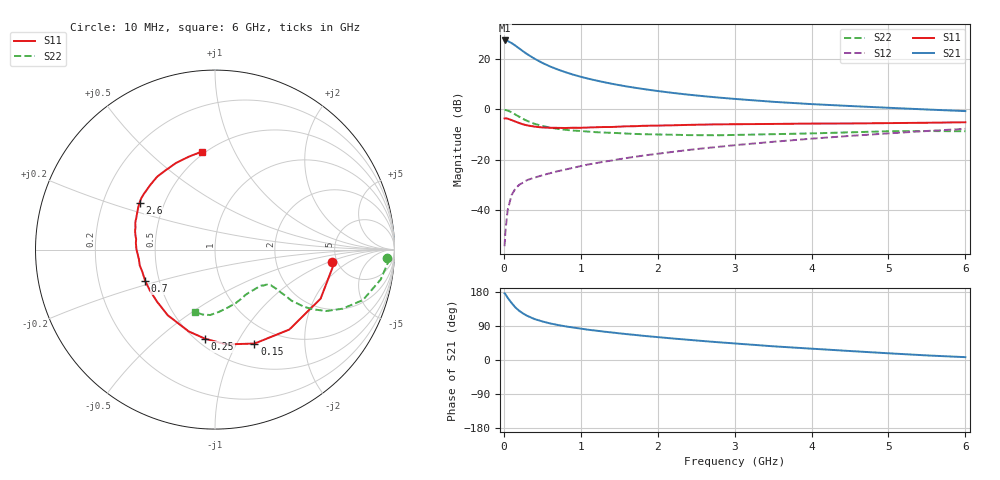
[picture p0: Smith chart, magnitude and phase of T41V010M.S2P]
! Infineon Technologies  Discrete & RF Semiconductors
! BFR182T
! Si NPN RF Bipolar Junction Transistor in SC75
! VCE = 1 V  IC = 10 mA
! Common Emitter S-Parameters:  October  1999
# GHz  S  MA  R  50
!  f  S11  S21  S12  S22
! GHz  MAG  ANG  MAG  ANG  MAG  ANG  MAG  ANG
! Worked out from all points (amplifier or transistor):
!   36 points, 10 MHz to 6 GHz, reference 50 ohm
!   highest |S21| = 27.3 dB at 10 MHz (marker M1)
!   |S21| within 3 dB of that: start of sweep to 192.3 MHz
!   unconditionally stable (mu >= 1): 760 MHz to 4.251 GHz
!   at 250 MHz: K = 0.51, MSG = 26.1 dB, |S12| = -29.1 dB
!   at 1.4 GHz: K = 1.16, MAG = 12.8 dB, |S12| = -20.4 dB
!   at 6 GHz: K = 0.90, MSG = 3.5 dB, |S12| = -7.8 dB
!   S11 on the Smith chart (normalised r, x): 10 MHz: 4.51, -1.12; 150 MHz: 0.77, -1.19; 250 MHz: 0.55, -0.73; 700 MHz: 0.42, -0.18; 2.6 GHz: 0.36, +0.25; 6 GHz: 0.48, +0.75
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0.01  0.6551 -6.2  23.23 176.0  0.0019 80.9  0.9588 -2.8
0.02  0.6621 -8.8  23.14 173.8  0.0037 92.6  0.9668 -4.2
0.05  0.6488 -24.9  22.64 164.2  0.01 80.3  0.9383 -10.2
0.1  0.6081 -47.1  20.66 150.6  0.0196 72.6  0.8711 -18.8
0.15  0.5679 -67.2  18.34 138.8  0.0265 63.9  0.7825 -24.9
0.2  0.5318 -83.2  16.12 129.8  0.0315 59.2  0.7081 -28.9
0.25  0.4999 -96.2  14.15 122.7  0.0349 56.0  0.6409 -31.3
0.3  0.4788 -107.8  12.52 116.9  0.0389 55.1  0.5899 -32.7
0.4  0.4508 -125.7  10.06 108.0  0.0438 54.3  0.5118 -33.7
0.5  0.434 -138.2  8.332 101.8  0.0486 55.1  0.4651 -33.2
0.6  0.4282 -148.3  7.073 96.6  0.0535 55.8  0.4322 -33.0
0.7  0.4262 -155.9  6.159 92.5  0.0586 57.3  0.4073 -32.6
0.9  0.4285 -168.3  4.869 85.7  0.0684 59.7  0.3762 -32.6
1.1  0.4331 -177.6  4.036 79.8  0.0799 61.7  0.3587 -33.4
1.3  0.4425 175.1  3.452 74.9  0.0907 62.6  0.3435 -34.8
1.6  0.458 166.5  2.83 68.2  0.1074 63.8  0.3278 -37.6
2.2  0.4795 154.7  2.106 56.7  0.1424 64.7  0.3111 -46.3
2.6  0.4951 148.1  1.813 49.9  0.1673 64.2  0.3047 -52.8
3.5  0.5098 134.9  1.404 36.2  0.2251 61.4  0.3192 -68.5
4.5  0.5208 121.7  1.158 23.7  0.295 56.1  0.3471 -86.1
5.5  0.5381 105.5  0.987 12.1  0.3694 49.7  0.3683 -100.9
6  0.5506 97.8  0.917 7.5  0.4073 45.6  0.365 -107.4
